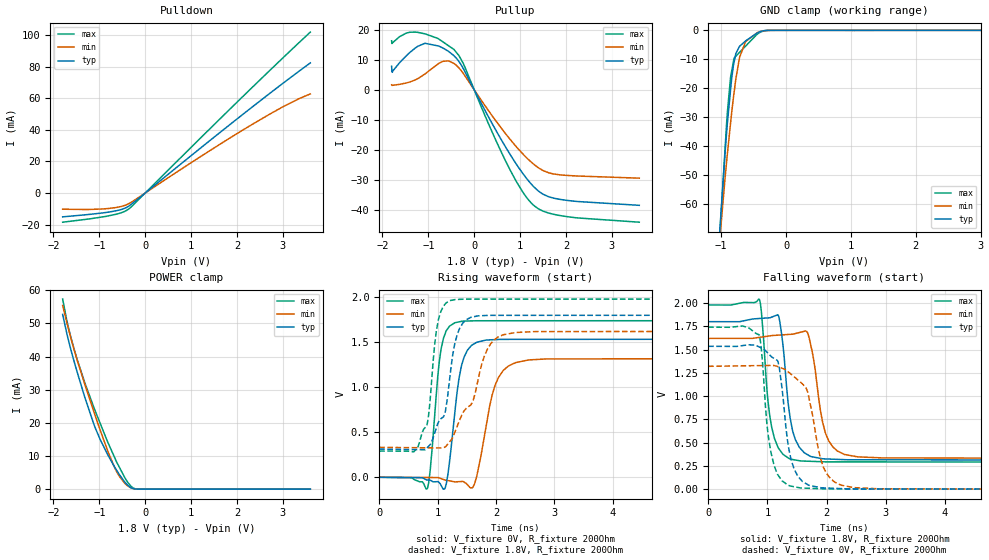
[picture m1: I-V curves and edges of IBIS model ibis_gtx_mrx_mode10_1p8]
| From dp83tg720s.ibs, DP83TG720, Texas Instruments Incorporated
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|   ibis_gtx_mrx_mode10_1p8
[Model]   ibis_gtx_mrx_mode10_1p8
Model_type   I/O
Polarity   Non-Inverting
Enable   Active-Low
Vinl = 0.54
Vinh = 1.26
Vmeas = 0.9
Vref = 0
Cref = 2pF
Rref = 100000
|   typ   min   max
C_comp   2.92pF   2.88pF   2.96pF
[Voltage Range]   1.8   1.62   1.98
[Temperature Range]   27   150   -40
[Pullup Reference]   1.8   1.62   1.98
[Pulldown Reference]   0   0   0
[Power Clamp Reference]   1.8   1.62   1.98
[GND Clamp Reference]   0   0   0
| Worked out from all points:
|   slope of the pulldown table from 0 to 0.27 V, typ, clamps not added: 42.1 ohm
|   slope of the pullup table from 0 to 0.27 V, typ, clamps not added: 34.5 ohm
|   GND clamp passes 1 mA (typ) near -0.45 V on its own axis
|   POWER clamp passes 1 mA (typ) near -0.37 V on its own axis
|   falling waveform, V_fixture 1.8V, R_fixture 200Ohm: 20-80 % time 163ps typ, 201ps min, 155ps max; typ from 1.8 V to 0.313 V
|   rising waveform, V_fixture 0V, R_fixture 200Ohm: 20-80 % time 177ps typ, 257ps min, 142ps max; typ from 0 V to 1.53 V
|   rising waveform, V_fixture 1.8V, R_fixture 200Ohm: 20-80 % time 289ps typ, 462ps min, 152ps max; typ from 0.313 V to 1.8 V
|   falling waveform, V_fixture 0V, R_fixture 200Ohm: 20-80 % time 188ps typ, 259ps min, 164ps max; typ from 1.53 V to 0 V
[Pulldown]
|   Voltage   I(typ)   I(min)   I(max)
-1.8V     -15.11mA   -10.25mA   -18.49mA
-1.222V   -13.57mA   -10.43mA   -16.42mA
-855mV    -12.34mA   -9.942mA   -14.81mA
-520.2mV  -10.44mA   -8.509mA   -12.5mA
-352.8mV  -8.213mA   -6.658mA   -9.977mA
1.165V    27.5mA     22.27mA    33.64mA
2.191V    51.23mA    40.99mA    62.89mA
3.06V     70.77mA    55.5mA     87.2mA
3.6V      82.43mA    62.79mA    101.9mA
[GND Clamp]
|   Voltage   I(typ)   I(min)   I(max)
-1.8V     -380.2mA   -330.5mA   -422.8mA
-1.017V   -67.69mA   -70.97mA   -69.38mA
-903.6mV  -31.87mA   -42.44mA   -28.15mA
-855mV    -20.52mA   -32.01mA   -16.18mA
-838.8mV  -16.74mA   -28.53mA   -14.19mA
-801mV    -11mA      -21.47mA   -9.556mA
-774mV    -8.056mA   -16.83mA   -8.932mA
-714.6mV  -5.478mA   -9.213mA   -7.557mA
-622.8mV  -3.648mA   -3.867mA   -5.433mA
-444.6mV  -916.7uA   -820uA     -1.31mA
-261mV    -11.9uA    -30.11uA   -11.43uA
3.6V      0A         0A         0A
[Pullup]
|   Voltage   I(typ)   I(min)   I(max)
-1.8V     7.801mA    1.623mA    16.26mA
-1.784V   5.785mA    1.465mA    15.52mA
-1.476V   11.34mA    2.257mA    18.84mA
-1.076V   15.41mA    5.196mA    18.59mA
-682.2mV  13.86mA    9.417mA    15.9mA
-444.6mV  11.35mA    8.796mA    13.42mA
-239.4mV  7.081mA    5.456mA    8.8mA
797.4mV   -21.84mA   -16.75mA   -27.06mA
1.051V    -27.63mA   -21.17mA   -33.8mA
1.31V     -32.4mA    -24.89mA   -38.57mA
1.845V    -36.36mA   -28.23mA   -41.73mA
3.6V      -38.41mA   -29.38mA   -44.01mA
[POWER Clamp]
|   Voltage   I(typ)   I(min)   I(max)
-1.8V     52.72mA    55.43mA    57.36mA
-1.681V   45.36mA    48.74mA    49.19mA
-1.546V   38.34mA    41.85mA    42.08mA
-1.319V   27.84mA    31.74mA    32.21mA
-1.082V   18.24mA    21.83mA    23.29mA
-979.2mV  14.91mA    17.7mA     19.75mA
-806.4mV  10.12mA    11.14mA    13.88mA
-612mV    5.438mA    5.014mA    7.891mA
-444.6mV  2.133mA    1.733mA    3.461mA
-293.4mV  326.9uA    316.9uA    674.2uA
-109.8mV  6.036uA    13.59uA    2.646uA
3.6V      0A         0A         0A
[Ramp]
R_load = 200
|   typ   min   max
dV/dt_r   0.920138/1.76785e-10   0.790833/2.54769e-10   1.04362/1.4137e-10
dV/dt_f   0.892229/1.62143e-10   0.772597/1.99067e-10   1.01338/1.52822e-10
[Falling Waveform]
V_fixture = 1.8V
V_fixture_min = 1.62V
V_fixture_max = 1.98V
R_fixture = 200Ohm
C_fixture = 0F
|   Time   V(typ)   V(min)   V(max)
0s        1.8V       1.62V      1.98V
865.1ps   1.834V     1.631V     2.04V
1.068ns   1.848V     1.65V      682.3mV
1.21ns    1.802V     1.656V     421.4mV
1.365ns   857.7mV    1.663V     330.3mV
1.475ns   529.1mV    1.673V     313.1mV
1.682ns   369.2mV    1.676V     300.3mV
1.974ns   325.4mV    619.8mV    293.7mV
2.302ns   317.3mV    373.3mV    293.2mV
6ns       313mV      332.4mV    291.1mV
[Rising Waveform]
V_fixture = 0V
V_fixture_min = 0V
V_fixture_max = 0V
R_fixture = 200Ohm
C_fixture = 0F
|   Time   V(typ)   V(min)   V(max)
0s        1.467uV    20.65uV    705.3nV
822.7ps   -29.69mV   -2.721mV   -128.2mV
1.055ns   -83.71mV   -13.63mV   1.404V
1.15ns    -71.39mV   -33.38mV   1.629V
1.291ns   691mV      -50.37mV   1.715V
1.51ns    1.41V      -82.19mV   1.736V
1.669ns   1.499V     4.289mV    1.739V
1.994ns   1.53V      1.036V     1.739V
2.335ns   1.532V     1.273V     1.739V
6ns       1.534V     1.318V     1.739V
[Rising Waveform]
V_fixture = 1.8V
V_fixture_min = 1.62V
V_fixture_max = 1.98V
R_fixture = 200Ohm
C_fixture = 0F
|   Time   V(typ)   V(min)   V(max)
0s        313mV      332.4mV    291.1mV
665.3ps   306.6mV    328.3mV    341.2mV
836ps     337.7mV    327.3mV    640.7mV
1.011ns   607.1mV    326.3mV    1.74V
1.127ns   715.2mV    336.1mV    1.923V
1.202ns   1.065V     390.8mV    1.961V
1.437ns   1.716V     719.1mV    1.978V
1.851ns   1.798V     1.42V      1.979V
2.119ns   1.799V     1.582V     1.979V
6ns       1.8V       1.62V      1.98V
[Falling Waveform]
|Gnd
V_fixture = 0V
V_fixture_min = 0V
V_fixture_max = 0V
R_fixture = 200Ohm
C_fixture = 0F
|   Time   V(typ)   V(min)   V(max)
0s        1.535V     1.32V      1.741V
862.3ps   1.529V     1.328V     1.659V
1.055ns   1.432V     1.33V      414.2mV
1.201ns   1.308V     1.311V     132.4mV
1.347ns   497.3mV    1.264V     44.04mV
1.592ns   83.18mV    1.131V     11.83mV
1.685ns   47.45mV    1.035V     9.615mV
1.942ns   13.86mV    245.3mV    3.514mV
2.243ns   5.995mV    43.93mV    2.263mV
6ns       1.608uV    20.63uV    743.6nV
